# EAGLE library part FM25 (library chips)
Cypress FRAM
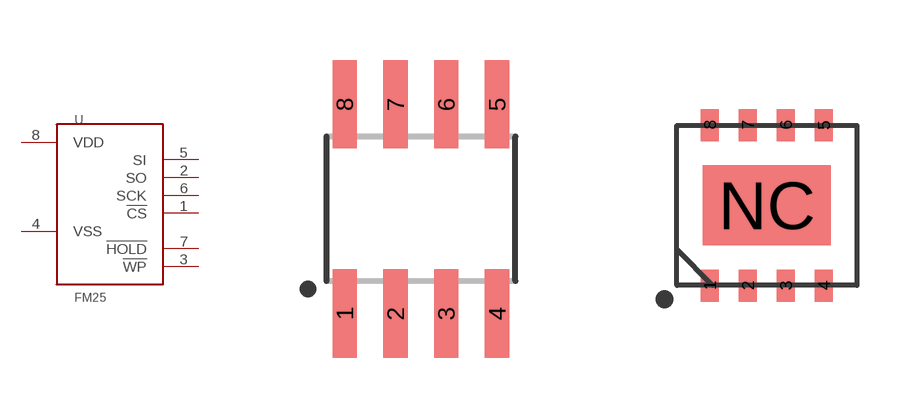
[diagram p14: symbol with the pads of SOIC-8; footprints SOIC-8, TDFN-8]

Designator prefix U

## FM25L04B-G (DIGIKEY: 428-3209-ND; MOUSER: 877-FM25L04B-G)  [SOIC-8]
1  !CS
2  SO
3  !WP
4  VSS
5  SI
6  SCK
7  !HOLD
8  VDD

## FM25L04B-DG (DIGIKEY: FM25L04B-DGRA-ND; MOUSER: 877-FM25L04B-DG)  [TDFN-8]
Pads as for SOIC-8

## FM25V20-DG (DIGIKEY: FM25V20-DGRA-ND; MOUSER: 877-FM25V20-DG)  [TDFN-8/6MM]
Pads as for SOIC-8

## FM25CLXXB-G  [SOIC-8]
Pads as for SOIC-8

## FM25CLXXB-DG  [TDFN-8]
Pads as for SOIC-8

## Footprint SOIC-8 (pad centres in mm)
smd 0.61 x 2.21: 1 -1.905,-2.616; 2 -0.635,-2.616; 3 0.635,-2.616; 4 1.905,-2.616; 5 1.905,2.616; 6 0.635,2.616; 7 -0.635,2.616; 8 -1.905,2.616

## Footprint TDFN-8 (pad centres in mm)
smd 0.45 x 0.8: 1 -1.425,-2.007; 2 -0.475,-2.007; 3 0.475,-2.007; 4 1.425,-2.007; 5 1.425,2.007; 6 0.475,2.007; 7 -0.475,2.007; 8 -1.425,2.007
smd 3.2 x 2: NC 0,0

## Footprint TDFN-8/6MM (pad centres in mm)
smd 0.55 x 1.2: 1 -1.905,-2.9; 2 -0.635,-2.9; 3 0.635,-2.9; 4 1.905,-2.9; 5 1.905,2.9; 6 0.635,2.9; 7 -0.635,2.9; 8 -1.905,2.9
smd 4 x 2.3: NC 0,0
